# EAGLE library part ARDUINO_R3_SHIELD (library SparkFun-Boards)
Arduino R3 Shield Footprint Shield form compatible with the Arduino Uno R3. SparkFun Products: MG2639 Cellular Shield MIDI Shield
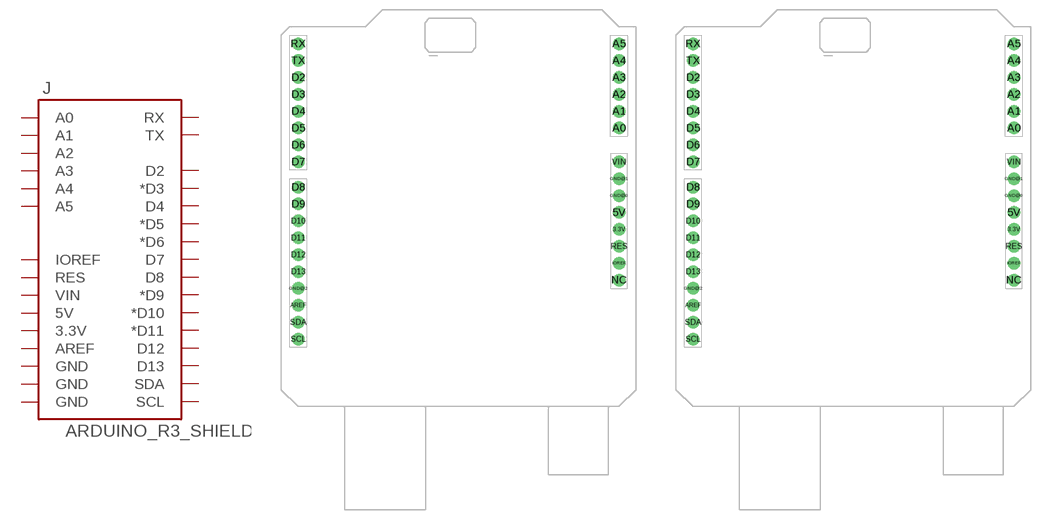
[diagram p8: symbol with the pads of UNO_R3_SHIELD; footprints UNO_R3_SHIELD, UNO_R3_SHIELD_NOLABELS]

Designator prefix J

## ARDUINO_R3_SHIELDBASIC  [UNO_R3_SHIELD]
3.3V  3.3V
5V  5V
A0  A0
A1  A1
A2  A2
A3  A3
A4  A4
A5  A5
AREF  AREF
D2  D2
D3  *D3
D4  D4
D5  *D5
D6  *D6
D7  D7
D8  D8
D9  *D9
D10  *D10
D11  *D11
D12  D12
D13  D13
GND@0  GND
GND@1  GND
GND@2  GND
IOREF  IOREF
RES  RES
RX  RX
SCL  SCL
SDA  SDA
TX  TX
VIN  VIN

## ARDUINO_R3_SHIELDNOLABELS  [UNO_R3_SHIELD_NOLABELS]
Pads as for UNO_R3_SHIELD

## ARDUINO_R3_SHIELDUNO_R3_SHIELD_LOCK  [UNO_R3_SHIELD_LOCK]
Pads as for UNO_R3_SHIELD

## ARDUINO_R3_SHIELDUNO_R3_SHIELD_NOLABELS_LOCK  [UNO_R3_SHIELD_NOLABELS_LOCK]
Pads as for UNO_R3_SHIELD

## Footprint UNO_R3_SHIELD (pad centres in mm)
Uno R3 Compatible Board Layout
drill 1.016 pad 1.88: 3.3V 50.8,26.67; 5V 50.8,29.21; A0 50.8,41.91; A1 50.8,44.45; A2 50.8,46.99; A3 50.8,49.53; A4 50.8,52.07; A5 50.8,54.61; AREF 2.54,15.24; D2 2.54,49.53; D3 2.54,46.99; D4 2.54,44.45; D5 2.54,41.91; D6 2.54,39.37; D7 2.54,36.83; D8 2.54,33.02; D9 2.54,30.48; D10 2.54,27.94; D11 2.54,25.4; D12 2.54,22.86; D13 2.54,20.32; GND@0 50.8,31.75; GND@1 50.8,34.29; GND@2 2.54,17.78; IOREF 50.8,21.59; NC 50.8,19.05; RES 50.8,24.13; RX 2.54,54.61; SCL 2.54,10.16; SDA 2.54,12.7; TX 2.54,52.07; VIN 50.8,36.83

## Footprint UNO_R3_SHIELD_NOLABELS (pad centres in mm)
drill 1.016 pad 1.88: 3.3V 50.8,26.67; 5V 50.8,29.21; A0 50.8,41.91; A1 50.8,44.45; A2 50.8,46.99; A3 50.8,49.53; A4 50.8,52.07; A5 50.8,54.61; AREF 2.54,15.24; D2 2.54,49.53; D3 2.54,46.99; D4 2.54,44.45; D5 2.54,41.91; D6 2.54,39.37; D7 2.54,36.83; D8 2.54,33.02; D9 2.54,30.48; D10 2.54,27.94; D11 2.54,25.4; D12 2.54,22.86; D13 2.54,20.32; GND@0 50.8,31.75; GND@1 50.8,34.29; GND@2 2.54,17.78; IOREF 50.8,21.59; NC 50.8,19.05; RES 50.8,24.13; RX 2.54,54.61; SCL 2.54,10.16; SDA 2.54,12.7; TX 2.54,52.07; VIN 50.8,36.83

## Footprint UNO_R3_SHIELD_LOCK (pad centres in mm)
Uno R3 Compatible Board Layout
drill 1.016 pad 1.88: 3.3V 50.8,26.67; 5V 51.054,29.21; A0 51.054,41.91; A1 50.8,44.45; A2 51.054,46.99; A3 50.8,49.53; A4 51.054,52.07; A5 50.8,54.61; AREF 2.286,15.24; D2 2.54,49.53; D3 2.286,46.99; D4 2.54,44.45; D5 2.286,41.91; D6 2.54,39.37; D7 2.286,36.83; D8 2.54,33.02; D9 2.286,30.48; D10 2.54,27.94; D11 2.286,25.4; D12 2.54,22.86; D13 2.286,20.32; GND@0 50.8,31.75; GND@1 51.054,34.29; GND@2 2.54,17.78; IOREF 50.8,21.59; NC 51.054,19.05; RES 51.054,24.13; RX 2.54,54.61; SCL 2.54,10.16; SDA 2.54,12.7; TX 2.286,52.07; VIN 50.8,36.83

## Footprint UNO_R3_SHIELD_NOLABELS_LOCK (pad centres in mm)
Uno R3 Compatible Board Layout
drill 1.016 pad 1.88: 3.3V 50.8,26.67; 5V 51.054,29.21; A0 51.054,41.91; A1 50.8,44.45; A2 51.054,46.99; A3 50.8,49.53; A4 51.054,52.07; A5 50.8,54.61; AREF 2.286,15.24; D2 2.54,49.53; D3 2.286,46.99; D4 2.54,44.45; D5 2.286,41.91; D6 2.54,39.37; D7 2.286,36.83; D8 2.54,33.02; D9 2.286,30.48; D10 2.54,27.94; D11 2.286,25.4; D12 2.54,22.86; D13 2.286,20.32; GND@0 50.8,31.75; GND@1 51.054,34.29; GND@2 2.54,17.78; IOREF 50.8,21.59; NC 51.054,19.05; RES 51.054,24.13; RX 2.54,54.61; SCL 2.54,10.16; SDA 2.54,12.7; TX 2.286,52.07; VIN 50.8,36.83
